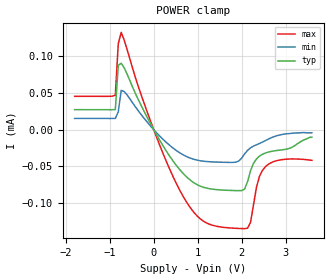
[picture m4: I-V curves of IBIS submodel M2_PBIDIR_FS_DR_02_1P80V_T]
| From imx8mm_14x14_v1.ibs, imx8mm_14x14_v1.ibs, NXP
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| Submodel
[Submodel]  M2_PBIDIR_FS_DR_02_1P80V_T
Submodel_type Dynamic_clamp
[POWER Clamp]
| Voltage   I(typ)   I(min)   I(max)
-1.8V     27.25uA    15.32uA    45.47uA
-874.1mV  27.29uA    15.35uA    46.98uA
-806.9mV  87.65uA    24.28uA    117.2uA
-739.7mV  90.49uA    53.55uA    132.5uA
-134.5mV  15.09uA    9.3uA      21.9uA
496.6mV   -47.21uA   -27.59uA   -71.03uA
931mV     -72.95uA   -40.65uA   -113.8uA
1.366V    -81.24uA   -43.97uA   -130.6uA
2.136V    -70.72uA   -28.14uA   -134.2uA
2.405V    -36.12uA   -18.82uA   -63.88uA
2.54V     -31.82uA   -15.02uA   -50.55uA
3.6V      -10.12uA   -4.292uA   -41.74uA
